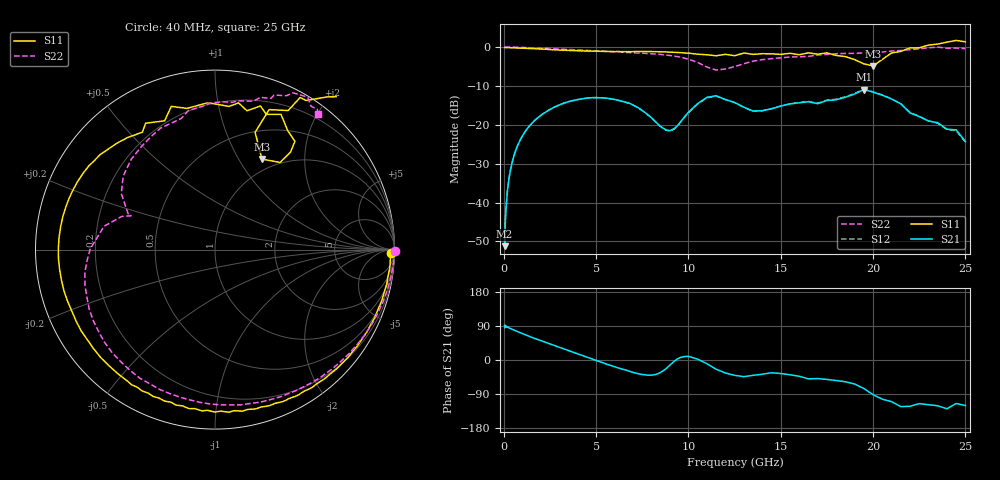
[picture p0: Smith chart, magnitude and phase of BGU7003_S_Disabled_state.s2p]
! Filename:  P:\Prog\Test\Noise\ATS_data\Testdata_Net\BGU7002 BGU7003 RN20082092\BGU7003_B1_high freq_off state_D.s2p
! Date/Time: Tue 16/Sep/2008 09:25:50
! BGU7003_B1_high freq_off state_R
! bias mode 0: Vout= 0.0000 V, Iout= 0.0000 mA, Vin= 0.0000 V, Iin= 0.0000 mA
! Date/time Wed Aug 13 12:34:14 2008
! Device data file deembeded for feedlines and parallel
! Original file: \BGU7002 BGU7003 RN20082092\BGU7003_B1_high freq_off state_R.s2p
! Feed-files: PR029V01_high frequency_140808_Feed1.s2p, PR029V01_high frequency_140808_Feed2.s2p
! Parallel-file: PR029V01_high frequency_140808_Par.s2p
# MHz S MA R 50
!  Freq-MHz  S11-mag  S11-arg  S21-mag  S21-arg  S12-mag  S12-arg  S22-mag  S22-arg
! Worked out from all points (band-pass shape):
!   166 points, 40 MHz to 25 GHz, reference 50 ohm
!   highest |S21| = -10.99 dB at 19.5 GHz (marker M1); lowest = -51.2 dB at 40 MHz (marker M2)
!   |S21| within 3 dB of the highest: 3.597 GHz to 6.394 GHz (2.797 GHz wide, 56 % of centre); 17.37 GHz to 21.24 GHz (3.868 GHz wide, 20 % of centre)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
!   lowest |S11| = -4.9 dB at 20 GHz (marker M3), VSWR 3.63, Z = 42.3 + j63.1 ohm
!   |S11| at or under -10 dB: nowhere
!   |S22| runs from -6.0 to 0.0 dB; largest |S21 - S12| = 0.0054
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40  0.9801 -1.2  0.002746 90.3  0.002901 89.3  1 -0.6
120  0.978 -3.4  0.008556 87.7  0.00875 88.0  0.9987 -1.7
350  0.9756 -9.8  0.02554 83.2  0.02562 83.2  0.9961 -4.9
1000  0.963 -27.4  0.07155 69.8  0.07166 69.7  0.9853 -13.7
1850  0.9438 -49.5  0.1235 53.7  0.124 53.6  0.9682 -25.0
3000  0.9087 -78.5  0.1793 33.3  0.1798 33.0  0.9396 -40.5
3900  0.8976 -99.3  0.2082 17.8  0.2085 17.4  0.9165 -53.3
5200  0.8781 -128.0  0.2218 -4.6  0.2215 -5.1  0.8864 -73.6
7000  0.8722 -164.8  0.1786 -32.9  0.1779 -33.2  0.8409 -107.5
8600  0.8645 164.1  0.09096 -29.4  0.09015 -29.6  0.7942 -144.3
9600  0.8437 146.4  0.1112 7.4  0.1099 7.3  0.7355 -170.2
11000  0.7922 128.1  0.225 -9.8  0.2223 -9.4  0.5517 160.5
13000  0.834 107.0  0.168 -43.9  0.1671 -43.7  0.6086 149.1
16500  0.8393 72.4  0.197 -49.8  0.1993 -49.3  0.7547 104.4
18500  0.7499 53.6  0.2255 -57.4  0.2289 -57.7  0.8248 87.2
19500  0.6059 53.3  0.2823 -75.2  0.2866 -75.9  0.8389 81.3
20000  0.568 62.6  0.2624 -91.5  0.2646 -92.3  0.8514 76.3
21000  0.8361 68.9  0.2138 -109.8  0.2149 -110.4  0.8847 73.4
22000  0.9714 60.8  0.142 -122.1  0.144 -123.0  0.9221 69.1
23500  1.087 51.6  0.106 -120.8  0.1046 -122.9  0.9943 58.7
24500  1.211 39.7  0.08589 -114.8  0.08368 -114.6  0.9674 53.9
25000  1.162 30.1  0.06096 -120.1  0.05988 -118.9  0.948 52.8
